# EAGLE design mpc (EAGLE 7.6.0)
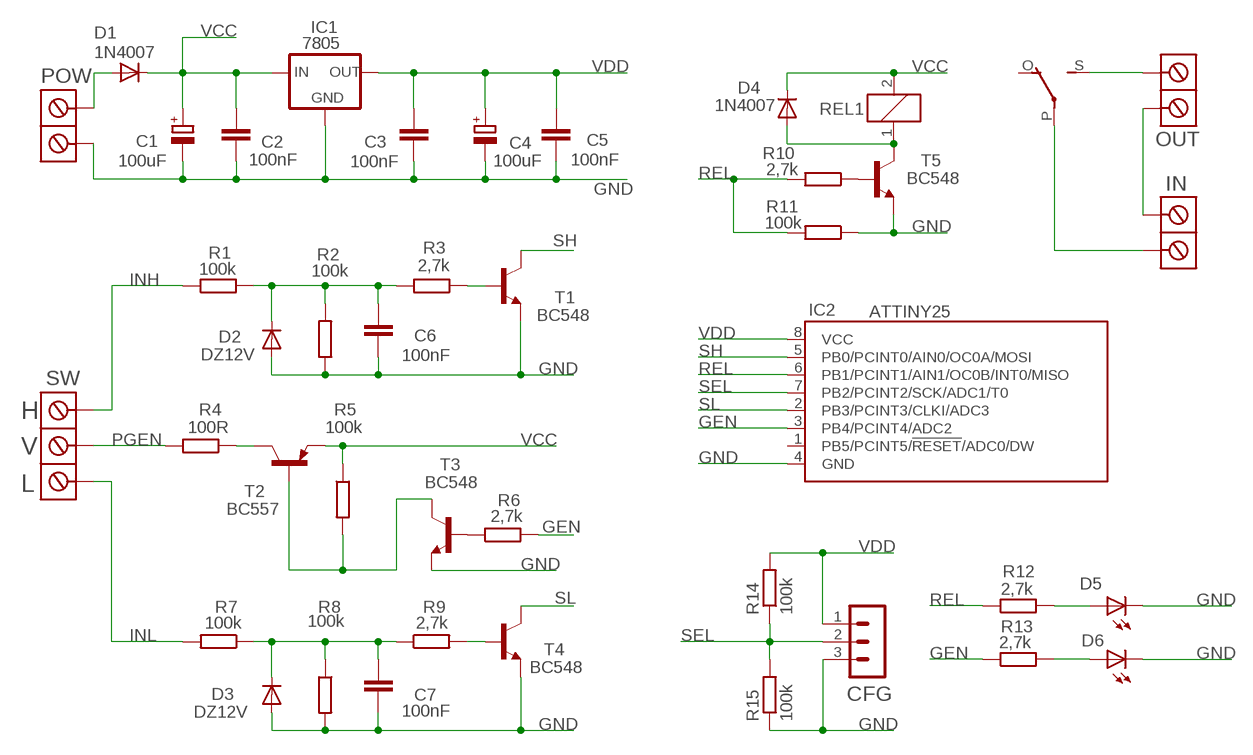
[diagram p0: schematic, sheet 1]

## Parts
C1  100uF  CPOL-EUE2.5-7  [E2,5-7]
C2  100nF  C-EU050-030X075  [C050-030X075]
C3  100nF  C-EU050-030X075  [C050-030X075]
C4  100uF  CPOL-EUE2.5-7  [E2,5-7]
C5  100nF  C-EU050-030X075  [C050-030X075]
C6  100nF  C-EU050-030X075  [C050-030X075]
C7  100nF  C-EU050-030X075  [C050-030X075]
CFG  MA03-1  [MA03-1]
D1  1N4007  1N4004  [DO41-10]
D2  DZ12V  1N4004  [DO41-10]
D3  DZ12V  1N4004  [DO41-10]
D4  1N4007  1N4004  [DO41-10]
D5  LED3MM  [LED3MM]
D6  LED3MM  [LED3MM]
IC1  7805  78LXX  [78LXX]
IC2  ATTINY25  TINY13-20PU  [DIL08]
IN  ARK2  [ARK2/750]
OUT  ARK2  [ARK2/750]
POW  ARK2ARK2/500  [ARK2/500]
R1  100k  R-EU_0207/7  [0207/7]
R2  100k  R-EU_0207/7  [0207/7]
R3  2,7k  R-EU_0207/7  [0207/7]
R4  100R  R-EU_0207/7  [0207/7]
R5  100k  R-EU_0207/7  [0207/7]
R6  2,7k  R-EU_0207/7  [0207/7]
R7  100k  R-EU_0207/7  [0207/7]
R8  100k  R-EU_0207/7  [0207/7]
R9  2,7k  R-EU_0207/7  [0207/7]
R10  2,7k  R-EU_0207/7  [0207/7]
R11  100k  R-EU_0207/7  [0207/7]
R12  2,7k  R-EU_0207/7  [0207/7]
R13  2,7k  R-EU_0207/7  [0207/7]
R14  100k  R-EU_0207/7  [0207/7]
R15  100k  R-EU_0207/7  [0207/7]
REL1  G5LE  [G5LE]
SW  ARK3ARK3/500  [ARK3/500]
T1  BC548  [TO92-EBC]
T2  BC557  [TO92-EBC]
T3  BC548  [TO92-EBC]
T4  BC548  [TO92-EBC]
T5  BC548  [TO92-EBC]

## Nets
GEN: IC2.3(PB4/PCINT4/ADC2) R6.2 R13.1
GND: C1.- C2.2 C3.2 C4.- C5.2 C6.2 C7.2 CFG.3 D2.A D3.A D5.K(C) D6.K(C) IC1.GND IC2.4(GND) POW.2 R2.1 R8.2 R11.1 R15.1 T1.E T3.E T4.E T5.E
INH: R1.1 SW.1
INL: R7.2 SW.3
N$1: R6.1 T3.B
N$3: D4.A REL1.1 T5.C
N$4: R10.1 T5.B
N$6: OUT.2 REL1.S(2:S)
N$7: IN.1 REL1.P(2:P)
N$8: D5.A R12.2
N$9: IN.2 OUT.1
N$10: R3.1 T1.B
N$11: D1.A POW.1
N$12: D6.A R13.2
N$13: C6.1 D2.C R1.2 R2.2 R3.2
N$14: R4.1 T2.C
N$15: R5.2 T2.B T3.C
N$19: R9.2 T4.B
N$21: C7.1 D3.C R7.1 R8.1 R9.1
PGEN: R4.2 SW.2
REL: IC2.6(PB1/PCINT1/AIN1/OC0B/INT0/MISO) R10.2 R11.2 R12.1
SEL: CFG.2 IC2.7(PB2/PCINT2/SCK/ADC1/T0) R14.1 R15.2
SH: IC2.5(PB0/PCINT0/AIN0/OC0A/MOSI) T1.C
SL: IC2.2(PB3/PCINT3/CLKI/ADC3) T4.C
VCC: C1.+ C2.1 D1.C D4.C IC1.IN R5.1 REL1.2 T2.E
VDD: C3.1 C4.+ C5.1 CFG.1 IC1.OUT IC2.8(VCC) R14.2
Unconnected: IC2.1(PB5/PCINT5/!RESET!/ADC0/DW) REL1.O(2:O)

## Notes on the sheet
- H
- V
- L

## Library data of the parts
C1 C4 = rcl:CPOL-EU: POLARIZED CAPACITOR, European symbol
C2 C3 C5-C7 = rcl:C-EU: CAPACITOR, European symbol
CFG = con-lstb:MA03-1: PIN HEADER; OC_FARNELL: unknown; OC_NEWARK: unknown
D1-D4 = diode:1N4004: DIODE
D5 D6 = led:LED: LED
IC1 = v-reg:78LXX: VOLTAGE REGULATOR
IC2 = atmel:TINY13: 8-bit AVR Microcontroller with 1K Bytes In-System Programmable Flash Source: http://www.atmel.com/dyn/resources/prod_documents/2535S.pdf; MPN: ATTINY13-20PU; OC_FARNELL: 9171550; OC_NEWARK: 96K6521
IN OUT POW = dimmer:ARK2
R1-R15 = rcl:R-EU_: RESISTOR, European symbol
REL1 = relay:G5LE: RELAY 1 x switch, 10 A/120 V AC, 8 A/30 V DC, Omron; OC_FARNELL: unknown; OC_NEWARK: unknown
SW = dimmer:ARK3
T1 T3-T5 = transistor-npn:BC548*: NPN Transistor
T2 = transistor-pnp:BC557*: PNP Transistror

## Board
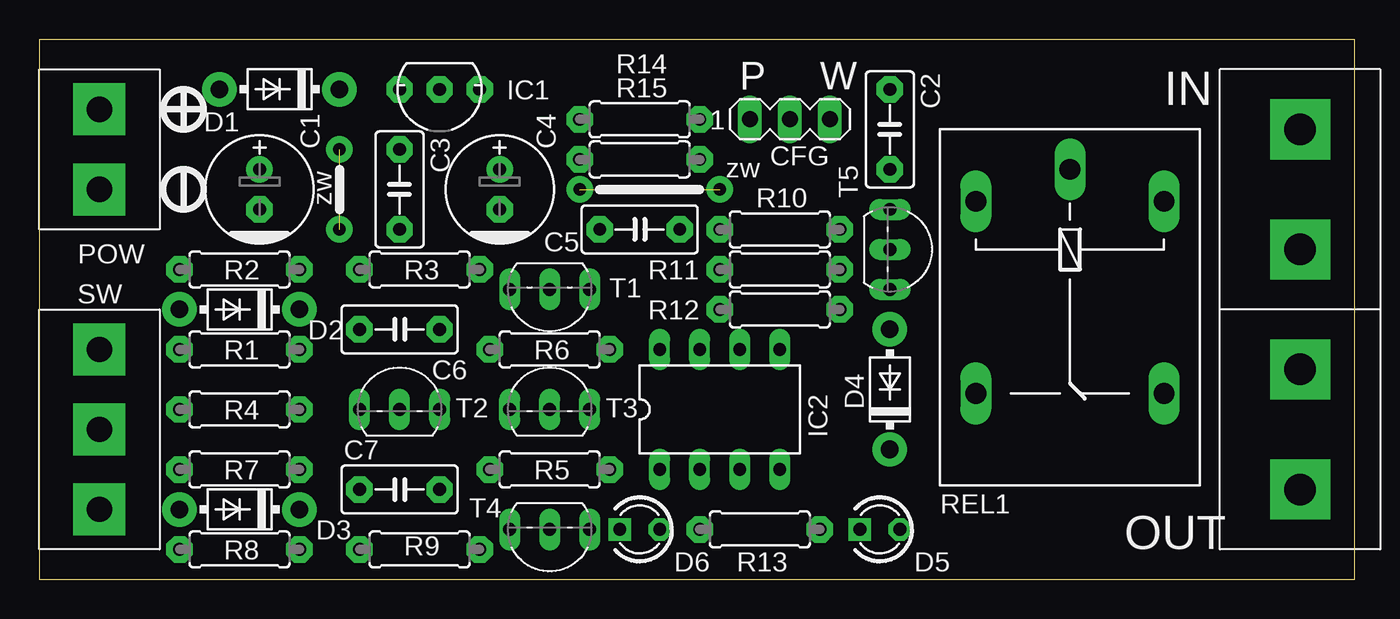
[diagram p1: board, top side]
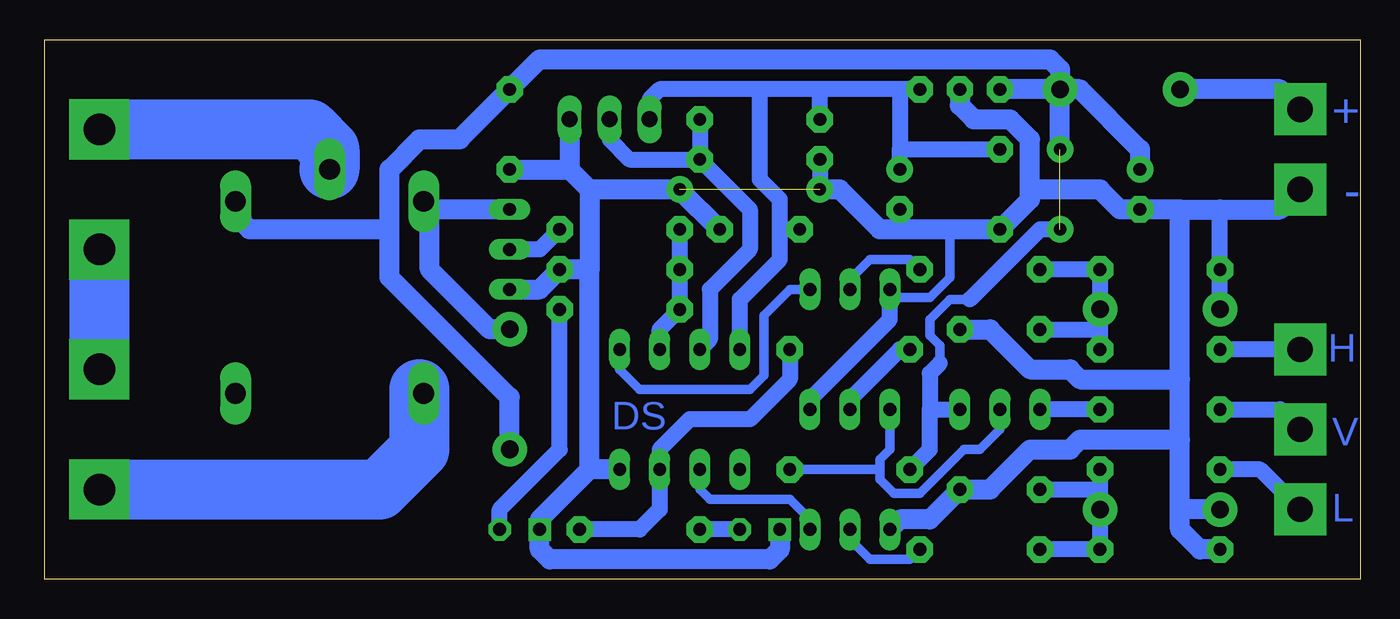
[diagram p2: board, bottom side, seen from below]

Size 83.49 x 34.28 mm. Coordinates in mm from the lower left corner, seen from the top.
Outline: 0,0 83.49,0 83.49,34.28 0,34.28 0,0
Copper layers (1*16): Top 0.035mm / dielectric 1.5mm / Bottom 0.035mm
Design rules "default": minimum track width 10mil, minimum drill 24mil, track to track 8mil, track to pad 8mil, pad to pad 8mil, via to via 8mil, smd to smd 8mil, copper to edge 40mil, drill to drill 8mil, minimum pad ring 10mil, minimum via ring 8mil, stop-mask expansion 4mil, vias tented up to drill 0mil, thermal gap 10mil

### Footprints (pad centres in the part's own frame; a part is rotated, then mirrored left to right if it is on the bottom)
E2,5-7 = drill 0.813 pad 1.676: + -1.27,0 | drill 0.813 pad 1.676 octagon: - 1.27,0
C050-030X075 = drill 0.813 pad 1.676 octagon: 1 -2.54,0; 2 2.54,0
MA03-1 = drill 1.016 long: 1 -2.54,0; 2 0,0; 3 2.54,0
DO41-10 = drill 1.118 pad 2.184: A 3.81,0; C -3.81,0
LED3MM = drill 0.813 pad 1.422 octagon: A -1.27,0 | drill 0.813 pad 1.422 square: K 1.27,0
78LXX = drill 0.813 pad 1.676 octagon: GND 0,0; IN 2.54,0; OUT -2.54,0
DIL08 = drill 0.813 long: 1 -3.81,-3.81; 2 -1.27,-3.81; 3 1.27,-3.81; 4 3.81,-3.81; 5 3.81,3.81; 6 1.27,3.81; 7 -1.27,3.81; 8 -3.81,3.81
ARK2/750 = drill 2 pad 3.81 square: 1 -3.81,0; 2 3.81,0
ARK2/500 = drill 1.6 pad 3.302 square: 1 -2.54,0; 2 2.54,0
0207/7 = drill 0.813 pad 1.676 octagon: 1 -3.81,0; 2 3.81,0
G5LE = drill 1.321 long: 1 -7.493,-5.969; 2 -7.493,5.969; O 4.699,5.969; P -9.525,0; S 4.699,-5.969
ARK3/500 = drill 1.6 pad 3.302 square: 1 -5.08,0; 2 0,0; 3 5.08,0
TO92-EBC = drill 0.813 long: B 0,-1.27; C -2.54,-1.27; E 2.54,-1.27

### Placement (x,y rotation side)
C1  13.97,24.76 270 top
C2  53.98,28.57 270 top
C3  22.86,24.76 270 top
C4  29.21,24.76 270 top
C5  38.1,22.22 0 top
C6  22.86,15.88 0 top
C7  22.86,5.71 0 top
CFG  47.62,29.21 0 top
D1  15.24,31.11 180 top
D2  12.7,17.14 180 top
D3  12.7,4.45 180 top
D4  53.98,12.06 90 top
D5  53.34,3.17 180 top
D6  38.1,3.17 180 top
IC1  25.4,31.11 180 top
IC2  43.18,10.79 0 top
IN  80.01,24.76 270 top
OUT  80.01,9.53 270 top
POW  3.81,27.3 270 top
R1  12.7,14.61 0 top
R2  12.7,19.68 0 top
R3  24.13,19.68 180 top
R4  12.7,10.79 180 top
R5  32.38,6.99 0 top
R6  32.38,14.61 0 top
R7  12.7,6.99 180 top
R8  12.7,1.91 180 top
R9  24.13,1.91 0 top
R10  46.99,22.22 180 top
R11  46.99,19.68 180 top
R12  46.99,17.14 0 top
R13  45.72,3.17 180 top
R14  38.1,29.21 180 top
R15  38.1,26.67 0 top
REL1  65.41,16.51 270 top
SW  3.81,9.53 270 top
T1  32.38,17.14 180 top
T2  22.86,12.06 0 top
T3  32.38,12.06 0 top
T4  32.38,1.91 180 top
T5  55.24,20.95 270 top

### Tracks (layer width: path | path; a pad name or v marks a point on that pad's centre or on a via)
GEN
  Bottom 1.016: R6.2 36.2,12.7 38.73,10.16 42.55,10.16 44.45,8.26 IC2.3 44.45,4.45 45.72,3.17 R13.1
GND  (via drill 0.8 pad 1.68)  (1 unrouted)
  Bottom 0.61: T1.E 29.97,18.41 29.97,17.91 27.3,17.91 26.04,19.18 26.04,22.22
  Bottom 1.016: D2.A R2.1 8.89,23.49 | T3.E 34.92,11.43 29.84,16.51 T1.E | R15.1 v34.29,24.76
  Bottom 1.27: 11.43,23.49 8.89,23.49 5.08,23.49 POW.2 | IC1.GND 25.4,30.1 24.51,29.21 22.23,29.21 20.95,27.94 20.95,24.76 | D3.A 11.43,4.45 | 11.43,4.45 11.43,8.89 | 11.43,8.89 11.43,12.7 | 11.43,12.7 11.43,23.49 | R8.2 10.16,1.91 11.43,3.17 11.43,4.45 | 11.43,8.89 17.78,8.89 18.41,8.26 20.95,8.26 23.5,5.71 C7.2 27.3,3.81 29.21,3.81 T4.E | C6.2 23.5,15.88 20.95,13.34 18.41,13.34 17.78,12.7 11.43,12.7 | 11.43,23.49 C1.- 15.24,23.49 16.51,24.76 20.95,24.76 | 20.95,24.76 20.95,24.13 C3.2 26.04,22.22 29.21,22.22 | C4.- 29.21,22.22 | 48.9,24.76 48.9,19.68 | 48.9,19.68 R11.1 52.07,18.41 T5.E | 48.9,24.76 v43.18,24.76 C5.2 | IC2.4 48.9,6.99 | 48.9,6.99 48.9,19.68 | 29.21,22.22 30.48,22.22 33.02,24.76 v34.29,24.76 | C2.2 50.16,26.04 | 50.16,26.04 48.9,24.76 | CFG.3 50.16,26.04 | D6.K 36.83,1.91 37.47,1.27 51.44,1.27 52.07,1.91 D5.K 52.07,3.81 48.9,6.99
INH
  Bottom 1.016: SW.1 R1.1
INL
  Bottom 1.016: SW.3 6.35,6.99 R7.2
N$1
  Bottom 1.016: T3.B 32.38,11.43 29.21,14.61 R6.1
N$3
  Bottom 1.016: 59.05,23.37 58.93,23.49
  Bottom 1.27: T5.C 58.93,23.49 REL1.1 | D4.A 55.24,15.88 59.05,19.68 59.05,23.37
N$4
  Bottom 1.016: R10.1 52.07,20.95 T5.B
N$6
  Bottom 2.54: 59.69,12.7 59.69,12.06 REL1.S
  Bottom 3.81: OUT.2 62.23,5.71 59.69,8.26 59.69,12.06
N$7
  Bottom 2.54: 65.41,25.4 REL1.P
  Bottom 3.81: IN.1 66.67,28.57 65.41,27.3 REL1.P
N$8
  Bottom 1.016: D5.A 54.61,4.45 50.8,8.26 R12.2
N$9
  Bottom 3.81: IN.2 OUT.1
N$10
  Bottom 0.61: T1.B 32.38,19.05 31.11,20.32 28.57,20.32 R3.1
N$11
  Bottom 1.27: POW.1 5.08,31.11 D1.A
N$12
  Bottom 1.016: D6.A R13.2
N$13
  Bottom 1.016: 16.51,15.88 D2.C R2.2 R3.2 | 16.51,15.88 R1.2 | C6.1 16.51,15.88
N$14
  Bottom 1.016: R4.1 T2.C
N$15
  Bottom 0.61: T2.B 22.86,9.53 24.13,8.26 25.15,8.26 27.94,5.46 29.59,5.46 30.48,6.35 30.48,6.99 | 30.48,6.99 30.48,7.62 29.84,8.26 T3.C | R5.2 30.48,6.99
N$19
  Bottom 0.61: T4.B 32.38,2.54 31.11,1.27 28.57,1.27 R9.2
N$21
  Bottom 1.016: R7.1 16.51,5.71 | 16.51,5.71 D3.C R8.1 R9.1 | C7.1 16.51,5.71
PGEN
  Bottom 1.016: R4.2 5.08,10.79 SW.2
REL
  Bottom 1.016: R10.2 R11.2 R12.1 44.45,15.88 IC2.6
SEL
  Bottom 1.016: CFG.2 47.62,27.94 46.35,26.67 R15.2 | R14.1 R15.2 | R15.2 38.73,23.49 38.73,20.95 41.27,18.41 41.27,15.24 IC2.7
SH
  Bottom 0.61: IC2.5 46.99,13.34 45.72,12.06 38.73,12.06 37.85,12.95 37.85,16.76 36.2,18.41 T1.C
SL
  Bottom 0.61: IC2.2 41.91,5.71 41.27,5.08 36.2,5.08 34.92,3.81 T4.C
VCC  (via drill 0.8 pad 1.68)  (1 unrouted)
  Bottom 0.61: 24.77,17.78 26.04,17.78 27.3,16.51 27.3,15.49 26.67,14.86 26.67,13.72
  Bottom 1.016: 26.67,13.72 27.3,13.08 27.3,10.79 | 27.3,10.79 T2.E | v19.05,22.22 20.32,22.22 24.77,17.78 | R5.1 27.3,8.26 27.3,10.79
  Bottom 1.27: D1.C IC1.IN | D1.C 17.78,31.11 13.97,27.3 C1.+ | v19.05,27.3 D1.C | D1.C 19.05,32.39 19.68,33.02 52.07,33.02 C2.1 57.15,27.94 59.69,27.94 61.59,26.04 61.59,22.22 | D4.C 53.98,11.56 61.59,19.18 61.59,22.22 | 61.59,22.22 70.48,22.22 71.12,22.86 71.12,23.75 REL1.2
VDD
  Bottom 1.016: C3.1 29.21,27.3 | C4.+ 29.21,27.3 | IC1.OUT 29.21,31.11 | 29.21,31.11 29.21,27.3 | 29.21,31.11 34.29,31.11 | 34.29,31.11 38.1,31.11 | 38.1,31.11 44.45,31.11 45.09,30.48 CFG.1 | R14.2 34.29,31.11 | IC2.8 39.37,17.78 36.83,20.32 36.83,22.22 | 36.83,22.22 36.83,24.13 38.1,25.4 38.1,31.11 | C5.1 36.83,22.22

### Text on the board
Bottom: + | - | H | DS | V | L
tPlace: P | W | zw | zw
